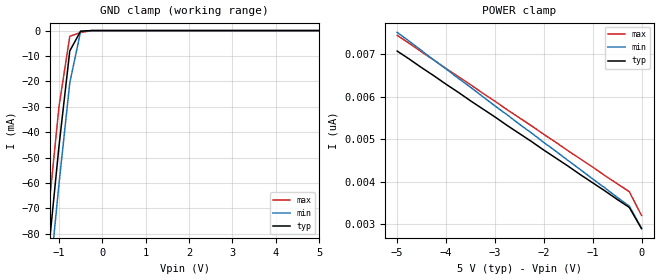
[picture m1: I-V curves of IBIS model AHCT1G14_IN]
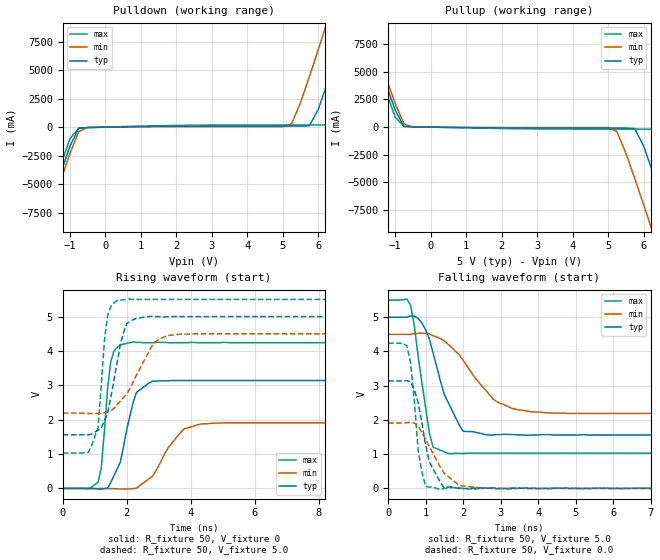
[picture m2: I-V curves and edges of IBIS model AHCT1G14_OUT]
| TEXAS INSTRUMENTS INCORPORATED
| Standard Linear and Logic Group
| IBIS Model of SN74AHCT1G14
| SINGLE SCHMITT-TRIGGER INVERTER
| SOT 5-pin (DCK) and SOT 5-pin (DBV) Package
[IBIS Ver]   3.2
[Comment Char]  |_char
[File Name]   ahct1g14.ibs
[File Rev]   2.0 J_die
[Date]   May 24, 2000
[Source]   Data created from HSPICE simulations at TI-SLL.
[Notes]   The following is an IBIS list for the AHCT1G14.
|   Please contact sllibis@ti.com with questions and
|   comments concerning SLL IBIS models.
[Disclaimer] Property of Texas Instruments Incorporated.  Unauthorized
   reproduction and/or distribution is strictly prohibited.
   This product is protected under copyright law.
   Created 2000, (C) Copyright 2000, Texas Instruments Inc.,
   All Rights Reserved.
   UNLESS THERE IS A SIGNED, WRITTEN AGREEMENT TO THE
   CONTRARY, TEXAS INSTRUMENTS () IS PROVIDING THE IBIS
   MODELS  AND WITHOUT ANY WARRANTY, EXPRESSED OR
   IMPLIED.  TI assumes no liability for:
   1) the accuracy of the IBIS models provided to your
   company;
   2) the proper functioning of these IBIS Models in your
   design or for any resulting applications; or
   3) infringement of patents, copyrights or intellectual
   property rights resulting from your use of these IBIS
   models.
   TI provides IBIS Models as a service to our customers.
   You and your company shall not distribute, sell or give
   these models to anyone else without prior written
   permission from TI.
   TI reserves the right to make changes to our products or
   to discontinue any semiconductor product or service
   without notice, and advises our customers to obtain the
   latest version of relevant information to verify, before
   placing orders, that the information being relied on is
   current.
   Please be aware that your receipt and use of the IBIS
   information provided shall serve as acceptance of these
   terms and conditions.  If you do not accept these terms,
   you should return or destroy the IBIS models and any
   other accompanying information immediately.
|   Component AHCT1G14_DCK
[Component]   AHCT1G14_DCK
[Manufacturer]  Texas Instruments, Inc.
[Package]
|   typ   min   max
R_pkg   0.020   0.017   0.025
L_pkg   0.998nH   0.881nH   1.069nH
C_pkg   0.146pF   0.118pF   0.205pF
[Pin]   signal_name   model_name   R_pin   L_pin   C_pin
1   NC   NC   0.019   1.069nH   0.162pF
2   A   AHCT1G14_IN   0.018   0.881nH   0.121pF
3   GND   GND   0.017   1.031nH   0.205pF
4   Y   AHCT1G14_OUT   0.020   0.960nH   0.124pF
5   VCC   POWER   0.025   1.049nH   0.118pF
|   Component AHCT1G14_DBV
[Component]   AHCT1G14_DBV
[Manufacturer]  Texas Instruments, Inc.
[Package]
|   typ   min   max
R_pkg   0.025   0.021   0.029
L_pkg   1.529nH   1.312nH   1.906nH
C_pkg   0.156pF   0.110pF   0.240pF
[Pin]   signal_name   model_name   R_pin   L_pin   C_pin
1   NC   NC   0.021   1.511nH   0.144pF
2   A   AHCT1G14_IN   0.023   1.312nH   0.138pF
3   GND   GND   0.029   1.906nH   0.240pF
4   Y   AHCT1G14_OUT   0.026   1.541nH   0.150pF
5   VCC   POWER   0.025   1.374nH   0.110pF
| Models and submodels in the file (2): AHCT1G14_IN (Input), AHCT1G14_OUT (Output)
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|   Model AHCT1G14_IN
[Model]   AHCT1G14_IN
Model_type  Input
Polarity   Inverting
Vinl = 0.8
Vinh = 2.0
| variable   typ   min   max
C_comp   1.24pf   0.93pf   1.55pf
[Temperature Range]   25   85   -40
[Voltage Range]   5.0   4.5   5.5
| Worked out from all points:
|   GND clamp passes 1 mA (typ) near -0.52 V on its own axis
[GND Clamp]
|   Voltage   I(typ)   I(min)   I(max)
-5V       -773mA     -786mA     -758mA
-1.5V     -133mA     -148mA     -117mA
-1.25V    -88.7mA    -104mA     -72.7mA
-1V       -45.6mA    -60.5mA    -30mA
-750mV    -7.99mA    -20.5mA    -2.23mA
-500mV    -233uA     -353uA     -759uA
-250mV    -2.63nA    -182nA     -26.9uA
5V        2.9nA      3.64nA     2.54nA
[POWER Clamp]
|   Voltage   I(typ)   I(min)   I(max)
-5V       7.08nA     7.52nA     7.45nA
-1.5V     4.37nA     4.5nA      4.73nA
-250mV    3.4nA      3.43nA     3.77nA
0V        2.9nA      2.91nA     3.21nA
|   Model AHCT1G14_OUT
[Model]   AHCT1G14_OUT
Model_type  Output
Polarity   Inverting
Vmeas = 2.50v
Cref = 15pf
| variable   typ   min   max
C_comp   3.12pf   2.34pf   3.90pf
[Temperature Range]   25   85   -40
[Voltage Range]   5.0   4.5   5.5
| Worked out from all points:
|   slope of the pulldown table from 0 to 0.75 V, typ, clamps not added: 18.8 ohm
|   slope of the pullup table from 0 to 0.75 V, typ, clamps not added: 25.3 ohm
|   rising waveform, R_fixture 50, V_fixture 0: 20-80 % time 473ps typ, 770ps min, 236ps max; typ from 0 V to 3.14 V
|   falling waveform, R_fixture 50, V_fixture 5.0: 20-80 % time 605ps typ, 1ns min, 343ps max; typ from 5 V to 1.56 V
|   rising waveform, R_fixture 50, V_fixture 5.0: 20-80 % time 422ps typ, 820ps min, 229ps max; typ from 1.56 V to 5 V
|   falling waveform, R_fixture 50, V_fixture 0.0: 20-80 % time 373ps typ, 610ps min, 218ps max; typ from 3.14 V to 0 V
[Pulldown]
|   Voltage   I(typ)   I(min)   I(max)
-5V       -40.9A     -41.4A     -40.3A
-1.75V    -8.76A     -9.39A     -8.09A
-1V       -1.69A     -2.33A     -1.02A
-750mV    -95.5mA    -395mA     -80.6mA
5.25V     93.4mA     298mA      192mA
5.75V     116mA      4.42A      192mA
6.25V     3.8A       9.19A      193mA
6.5V      6.17A      11.6A      931mA
6.75V     8.59A      14.1A      3.15A
7.25V     13.5A      19A        7.96A
7.5V      15.9A      21.4A      10.4A
10V       40.7A      46.2A      35.2A
[Pullup]
|   Voltage   I(typ)   I(min)   I(max)
-5V       40.7A      41.2A      40.1A
-2V       11A        11.6A      10.4A
-1.75V    8.59A      9.19A      7.96A
-1V       1.54A      2.14A      907mA
-750mV    63.6mA     284mA      62.5mA
5.25V     -84.4mA    -401mA     -178mA
5.75V     -130mA     -4.62A     -178mA
6.25V     -3.97A     -9.39A     -187mA
6.75V     -8.76A     -14.3A     -3.28A
7.25V     -13.6A     -19.2A     -8.09A
7.5V      -16.1A     -21.6A     -10.5A
10V       -40.9A     -46.4A     -35.3A
[Ramp]
| variable   typ   min   max
dV/dt_r   1.90E+00/4.50E-10   1.16E+00/7.61E-10   2.60E+00/2.51E-10
dV/dt_f   2.09E+00/5.57E-10   1.41E+00/1.02E-09   2.72E+00/3.52E-10
R_load = 50
[Rising Waveform]
R_fixture = 50
V_fixture = 0
|   Time   V(typ)   V(min)   V(max)
0s        0V         0V         0V
1.1ns     -16.6mV    -1.42mV    177mV
1.2ns     -21.9mV    -2.33mV    576mV
1.5ns     174mV      -6.39mV    3.7V
1.8ns     772mV      -13.8mV    4.18V
2.2ns     2.51V      -4.4mV     4.26V
2.8ns     3.12V      353mV      4.24V
3.7ns     3.14V      1.65V      4.24V
4.4ns     3.14V      1.88V      4.24V
25ns      3.14V      1.91V      4.24V
[Falling Waveform]
R_fixture = 50
V_fixture = 5.0
V_fixture_min = 4.5
V_fixture_max = 5.5
|   Time   V(typ)   V(min)   V(max)
0s        5V         4.5V       5.5V
600ps     5.04V      4.5V       5.35V
800ps     4.97V      4.53V      3.87V
1.1ns     4.37V      4.51V      1.62V
1.2ns     3.95V      4.46V      1.2V
1.6ns     2.52V      4.21V      1.02V
2ns       1.67V      3.74V      1.02V
2.9ns     1.57V      2.53V      1.03V
3.9ns     1.56V      2.23V      1.03V
25ns      1.56V      2.19V      1.03V
[Rising Waveform]
R_fixture = 50
V_fixture = 5.0
V_fixture_min = 4.5
V_fixture_max = 5.5
|   Time   V(typ)   V(min)   V(max)
0s        1.56V      2.19V      1.03V
800ps     1.56V      2.18V      1.05V
1.1ns     1.69V      2.18V      1.76V
1.3ns     1.97V      2.2V       4.29V
1.4ns     2.19V      2.23V      5.04V
1.7ns     3.68V      2.44V      5.47V
2ns       4.8V       2.75V      5.5V
2.8ns     5.01V      4.17V      5.5V
3.7ns     5V         4.49V      5.5V
25ns      5V         4.5V       5.5V
[Falling Waveform]
R_fixture = 50
V_fixture = 0.0
|   Time   V(typ)   V(min)   V(max)
0s        3.14V      1.91V      4.24V
500ps     3.15V      1.92V      4.17V
600ps     3.1V       1.93V      3.67V
800ps     2.51V      1.81V      1.12V
900ps     1.93V      1.63V      484mV
1.1ns     778mV      1.23V      34.4mV
1.3ns     366mV      817mV      -8.29mV
1.9ns     -5.42mV    85.8mV     11.3mV
2.8ns     -4.66mV    709uV      17.1mV
25ns      0V         0V         0V
